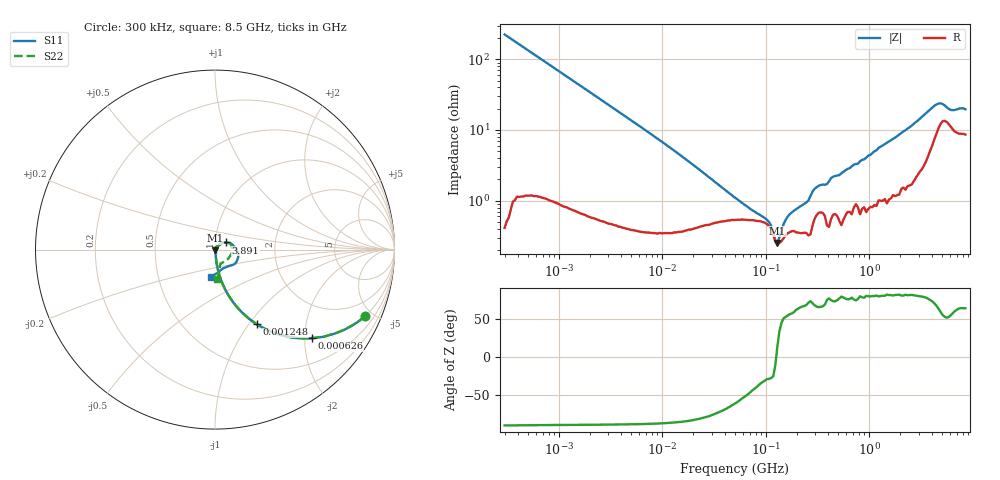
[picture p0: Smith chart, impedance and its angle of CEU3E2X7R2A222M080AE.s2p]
! S-parameter Generated by TDK Corporation
! Copyright(C) 2015 TDK Corporation.
! All Rights Reserved.
! TDK P/N: CEU3E2X7R2A222M080AE (Multilayer Ceramic Chip Capacitors)
! Property: C=2.2nF
! Size(LxWxT): 1.6x0.8x0.8mm, 0.063x0.031x0.031inches
! Model Type: s2p (Touchstone File Format Version 1.0)
! Frequency: DC=Yes Start=0.3MHz Stop=8500MHz 225points Log-sweep
! Note:
! Model Generated on Jun. 23, 2015
! Hash(MD5):
! Port Assignments:
!  1 ---| |--- 2
! Applicable Conditions:
!  Temperature = 25 degC
!  DC Bias Voltage = 0 V
!  Small Signal Operation
! Terms and conditions regarding TDK Simulation Models
! (1)This simulation model is being provided solely for informational purposes. Please refer to the specifications of the products in terms of detailed characteristics of such products.
! (2)In no event shall TDK Corporation of any of its subsidiaries be liable for any loss or damage arising, directly or indirectly,
!  From any information contained in this simulation model, including, but not limited to loss or damages arising from any inaccuracies, omissions or errors in connection with such information.
! (3)Any and all copyrights on this simulation model are owned by TDK Corporation.
!  Duplication or redistribution of this simulation model without prior written permission from TDK Corporation is prohibited.
! (4)This simulation model is subject to any modification or change without any prior notice.
! (5)Neither TDK Corporation nor any of its subsidiaries shall make any warranty, express or implied,
!  Including but not limited to the correctness, implied warranties of merchantability and fitness for a particular purpose with respect to this simulation models.
! (6)The use of this simulation model shall be deemed to have consented to the terms and conditions hereof.
# MHz S MA R 50
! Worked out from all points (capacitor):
!   224 points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, 300 kHz to 8.5 GHz, reference 50 ohm
!   read as one part in series: C = 2.35 nF near 314.1 kHz
!   lowest |Z| = 252 mohm at 129.6 MHz (marker M1)
!   series resonance near 126.5 MHz, so ESL is about 670 pH
!   S11 on the Smith chart (normalised r, x): 300 kHz: 1.00, -4.49; 626 kHz: 1.02, -2.17; 1.248 MHz: 1.02, -1.10; 3.891 GHz: 1.12, +0.09; 8.5 GHz: 0.92, -0.28
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0.3  0.9134 -24.0  0.4061 65.9  0.4067 66.0  0.9132 -24.1
0.6259918  0.7308 -42.4  0.673 47.0  0.6739 47.0  0.7308 -42.4
1.247529  0.4777 -60.6  0.8712 28.6  0.872 28.6  0.4776 -60.7
1.72111  0.3679 -67.5  0.9233 21.6  0.9243 21.6  0.3679 -67.5
9.430415  0.0718 -83.5  0.9932 4.1  0.9942 4.1  0.07173 -83.2
51.67171  0.0099 -77.0  0.993 0.4  0.9939 0.4  0.01498 -65.5
107.8202  0.004347 -75.8  0.9922 -0.1  0.9931 -0.1  0.009956 -80.9
129.5872  0.004198 -90.8  0.9944 -0.3  0.9954 -0.3  0.00481 -95.9
178.7805  0.002148 -130.5  0.9923 -0.8  0.9933 -0.8  0.002957 -54.9
235.5662  0.003307 -123.7  0.9911 -1.0  0.9921 -1.0  0.001086 -152.5
283.1228  0.00169 -49.2  0.9912 -1.3  0.992 -1.3  0.005203 93.1
373.0505  0.004252 37.1  0.9903 -1.7  0.9909 -1.7  0.002805 44.7
408.9767  0.002748 58.4  0.9923 -1.9  0.9932 -1.9  0.004053 73.5
448.3627  0.005227 66.2  0.9901 -2.2  0.991 -2.2  0.005253 31.1
514.6664  0.005675 86.0  0.9889 -2.4  0.9898 -2.4  0.001261 131.3
538.8791  0.003782 96.1  0.9899 -2.5  0.991 -2.5  0.004027 96.0
590.7752  0.002132 67.6  0.9879 -2.8  0.9888 -2.8  0.005262 78.9
710.042  0.004036 47.5  0.987 -3.3  0.988 -3.3  0.008499 56.5
893.5346  0.005322 35.7  0.9871 -4.1  0.988 -4.1  0.005826 53.7
1551.304  0.0131 50.5  0.9837 -7.1  0.9846 -7.1  0.01212 70.0
3890.506  0.07203 33.7  0.9412 -18.4  0.9419 -18.4  0.06922 36.2
8500  0.1521 -98.0  0.8917 -30.7  0.8933 -30.8  0.166 -85.7
